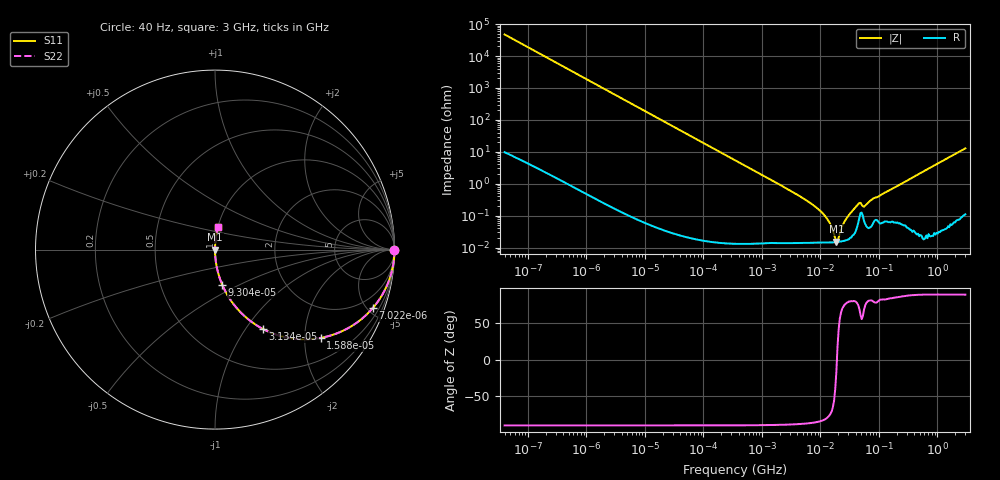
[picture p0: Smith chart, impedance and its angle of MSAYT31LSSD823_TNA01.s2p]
! MSAYT31LSSD823_TNA01  S-PARAMETER MODEL  ( General Type )
! Model Generated by TAIYO YUDEN Corporation (http://www.ty-top.com)
! Version 2.0
! TAIYO YUDEN Control No. 031016
! Copyright(c) 2003 TAIYO YUDEN CO.,LTD. All Rights Reserved.
! Product Description (link to TY-COMPAS)
! https://ds.yuden.co.jp/TYCOMPAS/or/detail?pn=MSAYT31LSSD823KTNA01&u=M
! Products Name : Multilayer Ceramic Capacitors
! Characteristics :
!  Capacitance : 0.082 uF , Rated Voltage : 25V
!  Case Size : 3.2 x 1.6 / 0.126 x 0.063 [mm/inch] , Thickness : 1.6 / 0.063 [mm/inch]
!  (Conditions: Temperature = 25 degC , DC Bias Current/Voltage = 0A / 0V)
! External Node Assignments :
!  1  o---| |---o  2
! GND o---------o GND
! Frequency Range : 40Hz  -  3GHz  [ 401 STEP ]
# MHz S RI R 50
! Freq[MHz].  S11 Real  S11 Imag  S21 Real  S21 Imag  S12 Real  S12 Imag  S22 Real  S22 Imag
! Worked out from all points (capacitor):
!   401 points, 40 Hz to 3 GHz, reference 50 ohm
!   read as one part in series: C = 83.9 nF near 44 Hz
!   lowest |Z| = 15.4 mohm at 18.71 MHz (marker M1)
!   series resonance near 19.11 MHz, so ESL is about 830 pH
!   S11 on the Smith chart (normalised r, x): 40 Hz: open; 7.022 kHz: 1.00, -5.40; 15.88 kHz: 1.00, -2.39; 31.34 kHz: 1.00, -1.21; 93.03 kHz: 1.00, -0.41; 3 GHz: 1.00, +0.26
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4e-05  1 -0.00211  4.88e-06 0.00211  4.88e-06 0.00211  1 -0.00211
0.000834  0.9981 -0.0439  0.00194 0.0439  0.00194 0.0439  0.9981 -0.0439
0.00271  0.98 -0.14  0.02 0.14  0.02 0.14  0.98 -0.14
0.007022  0.8794 -0.3256  0.1206 0.3256  0.1206 0.3256  0.8794 -0.3256
0.015879  0.5879 -0.492  0.4121 0.492  0.4121 0.492  0.5879 -0.492
0.017386  0.5434 -0.4979  0.4566 0.4979  0.4566 0.4979  0.5434 -0.4979
0.031343  0.2681 -0.4427  0.7319 0.4427  0.7319 0.4427  0.2681 -0.4427
0.093035  0.04 -0.1957  0.96 0.1957  0.96 0.1957  0.04 -0.1957
0.362475  0.00286 -0.0521  0.9971 0.0521  0.9971 0.0521  0.00286 -0.0521
7.222098  0.000146 -0.00225  0.9999 0.00225  0.9999 0.00225  0.000146 -0.00225
12.44272  0.000143 -0.000878  0.9999 0.000878  0.9999 0.000878  0.000143 -0.000878
14.91646  0.000144 -0.000488  0.9999 0.000488  0.9999 0.000488  0.000144 -0.000488
18.71131  0.000148 -4.22e-05  0.9999 4.22e-05  0.9999 4.22e-05  0.000148 -4.22e-05
20.48705  0.000151 0.000138  0.9998 -0.000138  0.9998 -0.000138  0.000151 0.000138
24.56009  0.00016 0.000517  0.9998 -0.000517  0.9998 -0.000517  0.00016 0.000517
28.13798  0.000172 0.000823  0.9998 -0.000823  0.9998 -0.000823  0.000172 0.000823
42.31378  0.000443 0.00205  0.9996 -0.00205  0.9996 -0.00205  0.000443 0.00205
46.32945  0.000875 0.00233  0.9991 -0.00233  0.9991 -0.00233  0.000875 0.00233
58.11596  0.000548 0.00198  0.9995 -0.00198  0.9995 -0.00198  0.000548 0.00198
79.8195  0.000601 0.0034  0.9994 -0.0034  0.9994 -0.0034  0.000601 0.0034
150.5692  0.000661 0.00617  0.9993 -0.00617  0.9993 -0.00617  0.000661 0.00617
3000  0.0172 0.1257  0.9828 -0.1257  0.9828 -0.1257  0.0172 0.1257
